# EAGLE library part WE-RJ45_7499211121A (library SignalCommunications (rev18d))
Order Code 7499211121A Design THT xBase-T 10/100 Base-T PoE Ports 1x1 Application PoE Tab Position DOWN LED (Left-Right) YELLOW-GREEN EMI Fingers Yes Details see: http://katalog.we-online.de/en/pbs/WE-LAN_RJ45/7499211121A? Updated by Yingchun Shan 2016-08-30 2016(C) Würth Elektronik
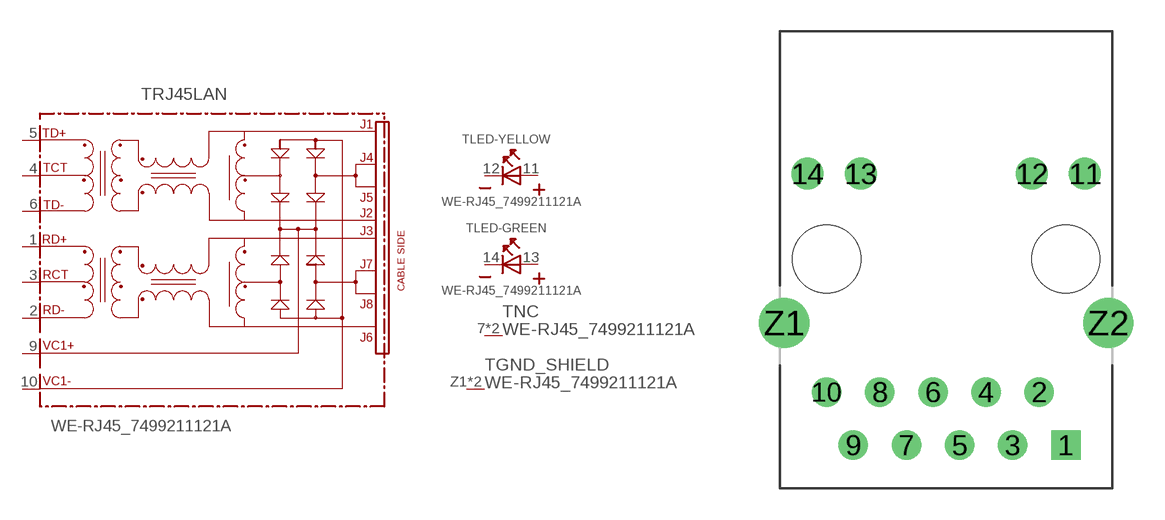
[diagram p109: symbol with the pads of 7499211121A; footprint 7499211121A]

Designator prefix T; gates LED-YELLOW=LED2PIN LED-GREEN=LED2PIN RJ45LAN=749921-THT-POE GND_SHIELD=GND_PIN NC=NC

## WE-RJ45_7499211121A (COMPANY-URL: http://www.we-online.de; CREATED-BY: Christin Zierenner; CREATED-DATE: AUG 2012; DATASHEET-URL: http://katalog.we-online.de/kataloge/eisos/media/pdf/7499211121A.pdf; MANUFACTURER: Würth Elektronik eiSos GmbH)  [7499211121A]
1  RJ45LAN:RD+
2  RJ45LAN:RD-  oc
3  RJ45LAN:RCT
4  RJ45LAN:TCT
5  RJ45LAN:TD+
6  RJ45LAN:TD-
7  NC:NC  nc
8  NC:NC  nc
9  RJ45LAN:VC1+  pwr
10  RJ45LAN:VC1-  pwr
11  LED-YELLOW:A  pas
12  LED-YELLOW:K  pas
13  LED-GREEN:A  pas
14  LED-GREEN:K  pas
Z1  GND_SHIELD:1  pwr
Z2  GND_SHIELD:1  pwr

## Footprint 7499211121A (pad centres in mm)
MAX HEIGHT=13.95mm PORTS----1X1 LED --YES
drill 0.9 square: 1 5.715,-8.89
drill 0.9: 2 4.445,-6.35; 3 3.175,-8.89; 4 1.905,-6.35; 5 0.635,-8.89; 6 -0.635,-6.35; 7 -1.905,-8.89; 8 -3.175,-6.35; 9 -4.445,-8.89; 10 -5.715,-6.35
drill 1.02: 11 6.63,4.08; 12 4.09,4.08; 13 -4.09,4.08; 14 -6.63,4.08
drill 1.6: Z1 -7.745,-3.05; Z2 7.745,-3.05
hole 3.25 at 5.715,0
hole 3.25 at -5.715,0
